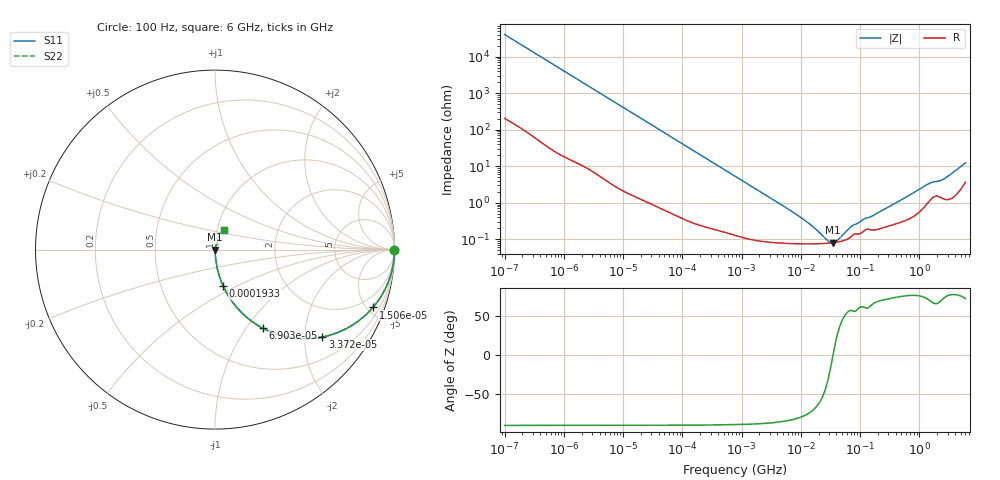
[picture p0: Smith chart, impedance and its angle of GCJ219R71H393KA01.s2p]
!Murata Part Number: GCJ219R71H393KA01
!These Parameters are Measured in Series Mode Connection
!Data Generated on Mar 13, 2026
!  o--ll--o
!Port1  Port2
!  o------o
!Operation Temp=25[degC], DC Bias Voltage=0[V]
!Freq. Start=100[Hz] Stop=6[GHz] 401[Steps]
# Hz S RI R 50
!Freq.(Hz) S11(Real) S11(Imag) S21(Real) S21(Imag) S12(Real) S12(Imag) S22(Real) S22(Imag)
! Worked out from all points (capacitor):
!   401 points, 100 Hz to 6 GHz, reference 50 ohm
!   read as one part in series: C = 39.3 nF near 109 Hz
!   lowest |Z| = 80.9 mohm at 34.83 MHz (marker M1)
!   series resonance near 34.87 MHz, so ESL is about 530 pH
!   S11 on the Smith chart (normalised r, x): 100 Hz: open; 15.06 kHz: 1.03, -5.45; 33.72 kHz: 1.02, -2.44; 69.03 kHz: 1.01, -1.20; 193.3 kHz: 1.00, -0.43; 6 GHz: 1.07, +0.24
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100  1 -0.00247  1.86e-05 0.00247  1.86e-05 0.00247  1 -0.00247
2008  0.9973 -0.0491  0.00267 0.0491  0.00267 0.0491  0.9973 -0.0491
5882  0.9791 -0.1404  0.0209 0.1404  0.0209 0.1404  0.9791 -0.1404
15062  0.8801 -0.322  0.1199 0.322  0.1199 0.322  0.8801 -0.322
22537  0.7677 -0.4192  0.2323 0.4192  0.2323 0.4192  0.7677 -0.4192
33721  0.5982 -0.4868  0.4018 0.4868  0.4018 0.4868  0.5982 -0.4868
40335  0.5109 -0.4963  0.4891 0.4963  0.4891 0.4963  0.5109 -0.4963
69028  0.2656 -0.4376  0.7344 0.4376  0.7344 0.4376  0.2656 -0.4376
112960  0.1208 -0.3213  0.8792 0.3213  0.8792 0.3213  0.1208 -0.3213
193316  0.0462 -0.2043  0.9538 0.2043  0.9538 0.2043  0.0462 -0.2043
361830  0.0148 -0.1132  0.9852 0.1132  0.9852 0.1132  0.0148 -0.1132
774597  0.00419 -0.0538  0.9958 0.0538  0.9958 0.0538  0.00419 -0.0538
6353432  0.00081 -0.00644  0.9992 0.00644  0.9992 0.00644  0.00081 -0.00644
1.555665e7  0.000757 -0.00218  0.9992 0.00218  0.9992 0.00218  0.000757 -0.00218
2.784235e7  0.000781 -0.000553  0.9992 0.000553  0.9992 0.000553  0.000781 -0.000553
3.482834e7  0.000808 -2.9e-06  0.9992 2.9e-06  0.9992 2.9e-06  0.000808 -2.9e-06
4.165952e7  0.000843 0.000437  0.9992 -0.000437  0.9992 -0.000437  0.000843 0.000437
7.455971e7  0.00129 0.00201  0.9987 -0.00201  0.9987 -0.00201  0.00129 0.00201
3.124326e8  0.0024 0.00756  0.9976 -0.00756  0.9976 -0.00756  0.0024 0.00756
1.369159e9  0.0105 0.0299  0.9895 -0.0299  0.9895 -0.0299  0.0105 0.0299
2.562649e9  0.0144 0.0413  0.9856 -0.0413  0.9856 -0.0413  0.0144 0.0413
6e9  0.0479 0.109  0.9521 -0.109  0.9521 -0.109  0.0479 0.109
